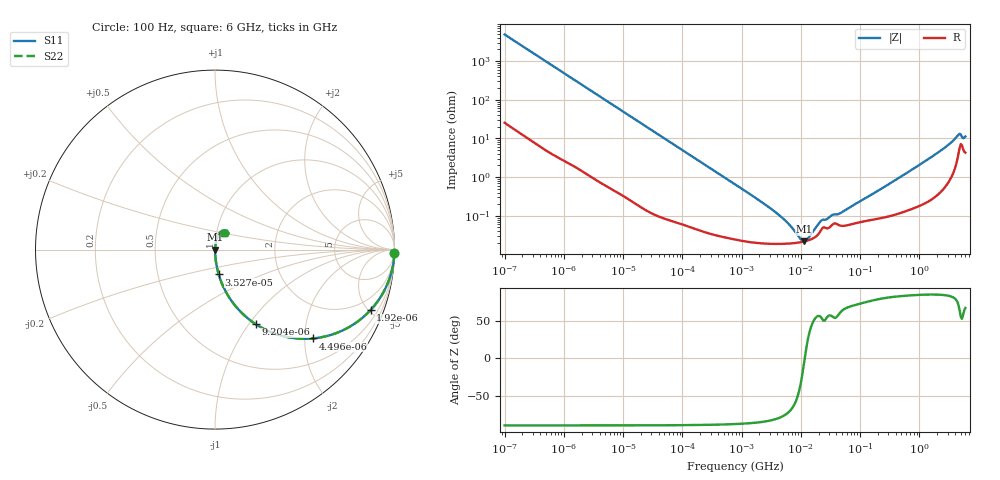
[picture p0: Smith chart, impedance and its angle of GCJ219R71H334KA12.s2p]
!Murata Part Number: GCJ219R71H334KA12
!These Parameters are Measured in Series Mode Connection
!Data Generated on Mar 13, 2026
!  o--ll--o
!Port1  Port2
!  o------o
!Operation Temp=25[degC], DC Bias Voltage=0[V]
!Freq. Start=100[Hz] Stop=6[GHz] 401[Steps]
# Hz S RI R 50
!Freq.(Hz) S11(Real) S11(Imag) S21(Real) S21(Imag) S12(Real) S12(Imag) S22(Real) S22(Imag)
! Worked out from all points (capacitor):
!   401 points, 100 Hz to 6 GHz, reference 50 ohm
!   read as one part in series: C = 326 nF near 109 Hz
!   lowest |Z| = 21.7 mohm at 11.37 MHz (marker M1)
!   series resonance near 11.65 MHz, so ESL is about 570 pH
!   S11 on the Smith chart (normalised r, x): 100 Hz: 2, -98; 1.92 kHz: 1.03, -5.13; 4.496 kHz: 1.01, -2.20; 9.204 kHz: 1.01, -1.08; 35.27 kHz: 1.00, -0.28; 6 GHz: 1.09, +0.21
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100  0.9995 -0.0205  0.000527 0.0205  0.000527 0.0205  0.9995 -0.0205
548  0.9871 -0.1102  0.0129 0.1102  0.0129 0.1102  0.9871 -0.1102
1920  0.8667 -0.337  0.1333 0.337  0.1333 0.337  0.8667 -0.337
2008  0.8561 -0.3481  0.1439 0.3481  0.1439 0.3481  0.8561 -0.3481
4496  0.5469 -0.4948  0.4531 0.4948  0.4531 0.4948  0.5469 -0.4948
9204  0.2263 -0.4152  0.7737 0.4152  0.7737 0.4152  0.2263 -0.4152
16473  0.0849 -0.2755  0.9151 0.2755  0.9151 0.2755  0.0849 -0.2755
35265  0.0205 -0.1382  0.9795 0.1382  0.9795 0.1382  0.0205 -0.1382
40335  0.0159 -0.1214  0.9841 0.1214  0.9841 0.1214  0.0159 -0.1214
774597  0.000286 -0.00652  0.9997 0.00652  0.9997 0.00652  0.000286 -0.00652
4246196  0.000189 -0.00104  0.9998 0.00104  0.9998 0.00104  0.000189 -0.00104
6353432  0.000192 -0.000566  0.9998 0.000566  0.9998 0.000566  0.000192 -0.000566
9941735  0.000208 -0.00014  0.9998 0.00014  0.9998 0.00014  0.000208 -0.00014
1.137099e7  0.000216 -2.1e-05  0.9998 2.1e-05  0.9998 2.1e-05  0.000216 -2.1e-05
1.300572e7  0.000229 9.87e-05  0.9998 -9.87e-05  0.9998 -9.87e-05  0.000229 9.87e-05
1.555665e7  0.000254 0.000264  0.9997 -0.000264  0.9997 -0.000264  0.000254 0.000264
2.225763e7  0.00044 0.000616  0.9996 -0.000616  0.9996 -0.000616  0.00044 0.000616
4.764863e7  0.000554 0.00106  0.9994 -0.00106  0.9994 -0.00106  0.000554 0.00106
3.124326e8  0.00102 0.00665  0.999 -0.00665  0.999 -0.00665  0.00102 0.00665
2.048624e9  0.00528 0.0423  0.9947 -0.0423  0.9947 -0.0423  0.00528 0.0423
4.385646e9  0.0391 0.1042  0.9609 -0.1042  0.9609 -0.1042  0.0391 0.1042
6e9  0.0506 0.0949  0.9494 -0.0949  0.9494 -0.0949  0.0506 0.0949
